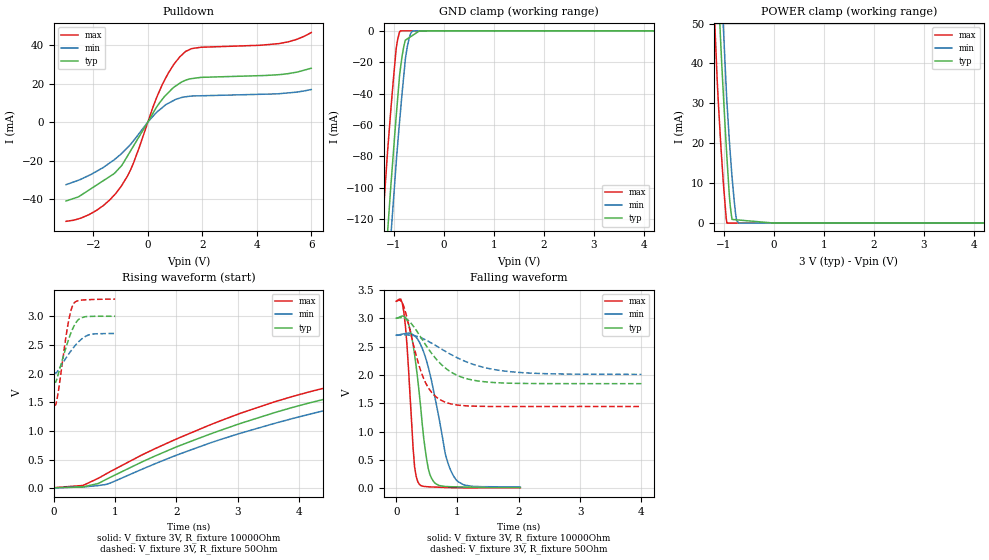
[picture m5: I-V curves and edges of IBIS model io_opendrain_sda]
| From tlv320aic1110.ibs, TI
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|   io_opendrain_sda Model
[Model]   io_opendrain_sda
Model_type   I/O_open_drain
Polarity   Non-Inverting
Enable   Active-Low
Vinl = 0.9
Vinh = 2.1
Vmeas = 1.5
Vref = 3.0
Cref = 15pF
Rref = 100000
|   typ   min   max
|   (nom PVT)   (Fast PVT)   (slow PVT)
|Average
C_comp   1.534e-12   1.442e-12   1.549e-12
|ON state : BUFFER OUTPUT TURNED HIGH
|C_comp (ON state)   5.555e-13   5.498e-13   5.491e-13
|OFF state: BUFFER IN HIGH IMPEDANCE
|C_comp (OFF state)   1.534e-12   1.442e-12   1.549e-12
| Where nom  PVT is Nominal Process,  3V,  65C
|   Fast PVT is Strong Process,   3.3V,  -40C
|   Slow PVT is Weak Process,   2.7V,  125C
[Model Spec]
|   typ   min   max
Vinl   0.9   0.81   0.99
Vinh   2.1   1.89   2.31
[Voltage Range]   3   2.7   3.3
|Ambient Temperature   25   105   -40
|Junction Temperature
[Temperature Range]   65   125   -40
[Pullup Reference]   3   2.7   3.3
[Pulldown Reference]   0   0   0
[Power Clamp Reference]   3   2.7   3.3
[GND Clamp Reference]   0   0   0
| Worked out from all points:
|   slope of the pulldown table from 0 to 0.45 V, typ, clamps not added: 43.4 ohm
|   GND clamp passes 1 mA (typ) near -0.54 V on its own axis
|   POWER clamp passes 1 mA (typ) near -0.84 V on its own axis
|   falling waveform, V_fixture 3V, R_fixture 10000Ohm: 20-80 % time 190ps typ, 297ps min, 112ps max; typ from 3 V to 0.011 V
|   rising waveform, V_fixture 3V, R_fixture 10000Ohm: 20-80 % time 8ns typ, 8.09ns min, 7.88ns max; typ from 0.005 V to 3 V
|   falling waveform, V_fixture 3V, R_fixture 50Ohm: 20-80 % time 519ps typ, 803ps min, 309ps max; typ from 3 V to 1.85 V
|   rising waveform, V_fixture 3V, R_fixture 50Ohm: 20-80 % time 206ps typ, 287ps min, 153ps max; typ from 1.85 V to 3 V
[Pulldown]
|   Voltage   I(typ)   I(min)   I(max)
-3V       -40.91mA   -32.43mA   -51.44mA
-1.888V   -32.73mA   -25.57mA   -45.83mA
-1.403V   -28.27mA   -21.23mA   -40.44mA
-990.3mV  -23.03mA   -16.66mA   -33.57mA
-534.9mV  -12.61mA   -9.865mA   -21.57mA
194.4mV   4.738mA    3.099mA    7.971mA
540.9mV   12mA       7.635mA    19.71mA
956.7mV   18.1mA     11.28mA    29.99mA
1.382V    21.72mA    13.12mA    36.59mA
1.943V    23.19mA    13.66mA    38.81mA
4.824V    24.63mA    14.74mA    40.74mA
6V        27.96mA    16.91mA    46.44mA
[GND Clamp]
-3V       -1.06A     -1.084A    -1.022A
-1.226V   -174.2mA   -206.2mA   -122.9mA
-1.129V   -129.1mA   -161mA     -77.5mA
-1.048V   -92.9mA    -124.6mA   -44.82mA
-954mV    -54.11mA   -83.69mA   -10.99mA
-868.2mV  -23.54mA   -51mA      0A
-804mV    -10.24mA   -28.92mA   0A
-767.1mV  -5.887mA   -16.97mA   0A
-696.9mV  -4.402mA   -4.903mA   0A
-632.1mV  -3.031mA   -128.2uA   0A
-489mV    -4.545uA   0A         0A
6V        0A         0A         0A
[POWER Clamp]
-3V       666.4mA    683.3mA    644.5mA
-1.239V   95.21mA    113.9mA    66.05mA
-1.175V   76.32mA    94.68mA    46.84mA
-1.135V   64.71mA    83.01mA    35.27mA
-1.071V   46.22mA    64.68mA    20.78mA
-1.013V   32.13mA    48.85mA    9.877mA
-942.6mV  16.4mA     30.31mA    0A
-894mV    6.831mA    20.6mA     0A
-840mV    897.2uA    11.53mA    0A
-769.8mV  822uA      2.408mA    0A
-707.7mV  755.4uA    0A         0A
6V        0A         0A         0A
[Ramp]
R_load = 10000
|   typ   min   max
dV/dt_r   1.79289/8.00016e-09   1.61053/8.07659e-09   1.97507/7.87534e-09
dV/dt_f   1.79333/1.8967e-10   1.61098/2.98349e-10   1.97547/1.11873e-10
[Falling Waveform]
V_fixture = 3V
V_fixture_min = 2.7V
V_fixture_max = 3.3V
R_fixture = 10000Ohm
|   Time   V(typ)   V(min)   V(max)
0s        3V         2.7V       3.3V
125ps     3.034V     2.726V     3.11V
175ps     2.972V     2.736V     2.538V
300ps     2.359V     2.689V     377.5mV
375ps     1.688V     2.585V     74.15mV
450ps     873.8mV    2.398V     33.65mV
550ps     241.2mV    2.02V      24.68mV
800ps     31.55mV    610.7mV    13.64mV
950ps     25.91mV    191mV      9.585mV
2.025ns   11.14mV    21.64mV    7.542mV
[Rising Waveform]
V_fixture = 3V
V_fixture_min = 2.7V
V_fixture_max = 3.3V
R_fixture = 10000Ohm
|   Time   V(typ)   V(min)   V(max)
0s        5.113mV    5.034mV    7.545mV
475ps     20.93mV    20.12mV    46.69mV
850ps     150.1mV    64.25mV    246.8mV
2.675ns   992.2mV    833.4mV    1.158V
4.7ns     1.622V     1.422V     1.816V
8.7ns     2.274V     2.014V     2.54V
12.85ns   2.664V     2.383V     2.949V
17.23ns   2.849V     2.557V     3.145V
23.2ns    2.948V     2.65V      3.248V
49.98ns   2.999V     2.699V     3.299V
[Falling Waveform]
V_fixture = 3V
V_fixture_min = 2.7V
V_fixture_max = 3.3V
R_fixture = 50Ohm
|   Time   V(typ)   V(min)   V(max)
0s        3V         2.7V       3.3V
75ps      3.012V     2.706V     3.309V
125ps     3.007V     2.706V     3.204V
350ps     2.751V     2.677V     2.249V
475ps     2.54V      2.621V     1.872V
600ps     2.349V     2.547V     1.665V
775ps     2.146V     2.434V     1.531V
1.15ns    1.934V     2.229V     1.454V
1.775ns   1.857V     2.068V     1.443V
4ns       1.846V     2.009V     1.442V
[Rising Waveform]
V_fixture = 3V
V_fixture_min = 2.7V
V_fixture_max = 3.3V
R_fixture = 50Ohm
|   Time   V(typ)   V(min)   V(max)
0s        1.846V     2.009V     1.442V
30ps      1.848V     2.011V     1.452V
50ps      1.909V     2.024V     1.54V
75ps      1.998V     2.065V     1.695V
225ps     2.544V     2.313V     2.824V
275ps     2.699V     2.389V     3.085V
325ps     2.821V     2.459V     3.225V
425ps     2.962V     2.576V     3.278V
575ps     2.995V     2.677V     3.29V
1ns       3V         2.7V       3.3V
